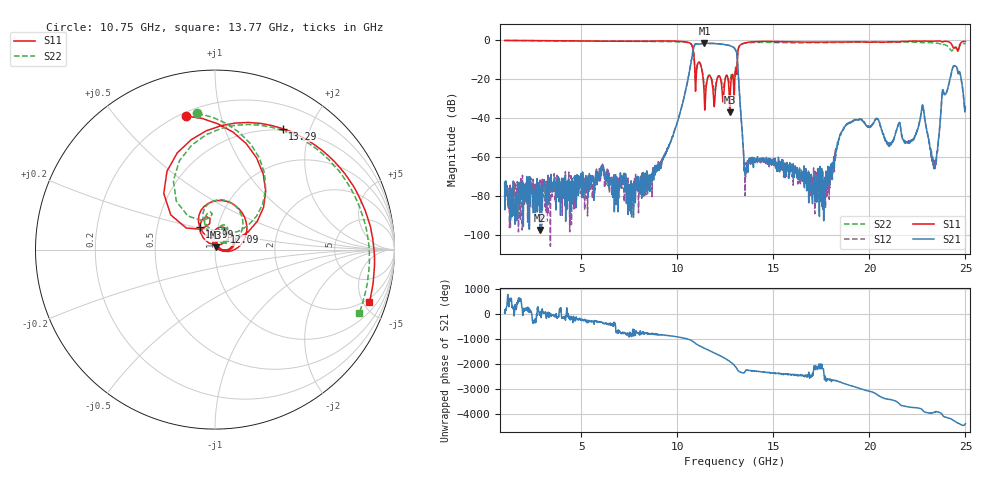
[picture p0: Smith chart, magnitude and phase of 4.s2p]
!The following data was pulled from an Agilent PNA
!This sNp file was generated from the data in the RF Test software
!NOTE:  Smoothing/Math/Corrections applied on any given trace ARE included in the data saved here
# MHz S dB R 50
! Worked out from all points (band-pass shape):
!   1601 points, 1 GHz to 25 GHz, reference 50 ohm
!   highest |S21| = -1.40 dB at 11.41 GHz (marker M1); lowest = -97.3 dB at 2.845 GHz (marker M2)
!   |S21| within 3 dB of the highest: 10.83 GHz to 13 GHz (2.168 GHz wide, 18.2 % of centre)
!   lowest |S11| = -36.9 dB at 12.73 GHz (marker M3), VSWR 1.03, Z = 50.4 + j1.38 ohm
!   |S11| at or under -10 dB: 10.88 GHz to 13.12 GHz (2.243 GHz wide, 18.7 % of centre)
!   |S22| runs from -25.5 to 0.0 dB; largest |S21 - S12| = 0.0066
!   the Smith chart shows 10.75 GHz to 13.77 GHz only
!   S11 on the Smith chart (normalised r, x): 10.75 GHz: 0.22, +0.78; 10.99 GHz: 0.82, +0.21; 12.09 GHz: 1.09, +0.21; 13.29 GHz: 0.48, +1.60; 13.77 GHz: 1.66, -5.54
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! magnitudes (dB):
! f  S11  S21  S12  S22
! 1 GHz  0.0  -72.8  -80.0  0.0
! 2.845 GHz  -0.1  -97.3  -71.7  -0.1
! 5.005 GHz  -0.3  -78.9  -73.5  -0.3
! 9.01 GHz  -0.3  -64.3  -62.2  -0.5
! 10.75 GHz  -2.4  -8.9  -8.8  -2.3
! 10.99 GHz  -16.4  -1.8  -1.8  -15.7
! 11.41 GHz  -31.3  -1.4  -1.4  -24.3
! 12.09 GHz  -19.2  -1.7  -1.7  -19.3
! 12.73 GHz  -36.9  -2.6  -2.6  -21.4
! 13 GHz  -17.8  -4.4  -4.4  -16.0
! 13.29 GHz  -2.2  -35.1  -35.1  -2.2
! 13.51 GHz  -1.3  -67.6  -67.9  -1.4
! 13.77 GHz  -0.8  -62.0  -60.0  -1.1
! 17 GHz  -0.9  -74.6  -70.2  -1.2
! 17.83 GHz  -0.8  -73.6  -67.5  -1.1
! 18.91 GHz  -0.8  -42.5  -42.3  -1.0
! 21.01 GHz  -0.7  -53.2  -53.7  -1.0
! 22.78 GHz  -0.4  -33.3  -33.4  -1.2
! 23.39 GHz  -0.4  -65.3  -62.7  -1.3
! 23.83 GHz  -0.7  -25.2  -25.5  -2.4
! 24.43 GHz  -3.8  -12.9  -13.0  -3.5
! 25 GHz  -0.5  -33.9  -34.3  -1.9
